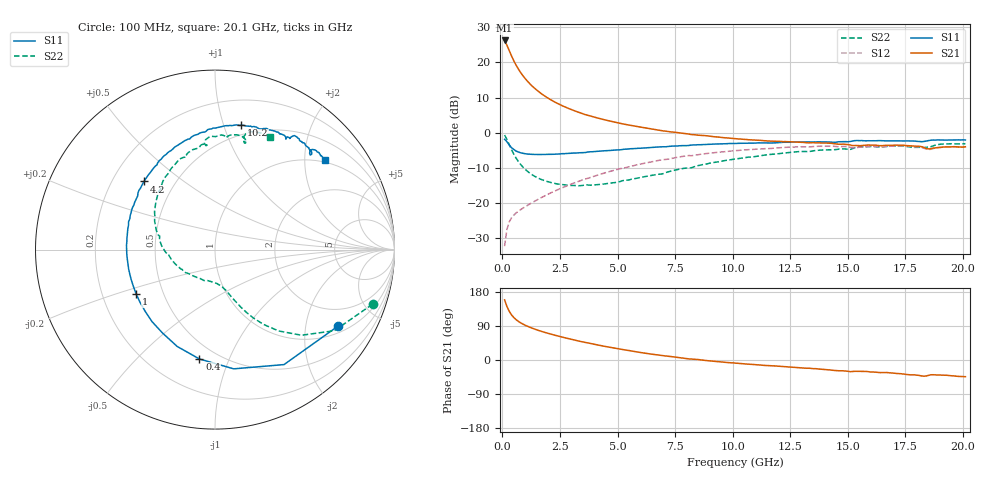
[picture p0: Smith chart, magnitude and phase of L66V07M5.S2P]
!  Infineon Technologies AG
! BFR380L3 , PF131585-7, No.6, Th 09.10.01, soldered on pcb-board, measured with PP GSG850
!  Vce=6.0 V,  Ic=7.5 mA
! Common Emitter S-Parameters:  15. November 2001
#  GHz  S  MA  R  50
! f  S11  S21  S12  S22
! GHz  Mag  Ang  Mag  Ang  Mag  Ang  Mag  Ang
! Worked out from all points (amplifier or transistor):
!   201 points, 100 MHz to 20.1 GHz, reference 50 ohm
!   highest |S21| = 26.2 dB at 100 MHz (marker M1)
!   |S21| within 3 dB of that: start of sweep to 307.7 MHz
!   unconditionally stable (mu >= 1): 2.049 GHz to 4.436 GHz
!   at 3.4 GHz: K = 1.04, MAG = 8.4 dB, |S12| = -13.6 dB
!   at 10.1 GHz: K = 0.93, MSG = 1.7 dB, |S12| = -5.1 dB
!   at 20.1 GHz: K = 0.99, MSG = 0.0 dB, |S12| = -4.0 dB
!   S11 on the Smith chart (normalised r, x): 100 MHz: 1.25, -3.05; 400 MHz: 0.40, -0.78; 1 GHz: 0.35, -0.23; 4.2 GHz: 0.34, +0.36; 10.2 GHz: 0.41, +1.14; 20.1 GHz: 0.95, +2.52
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0.1  0.8077 -31.8  20.44 158.5  0.02458 73.1  0.9288 -19.1
0.2  0.7472 -59.0  17.5 141.3  0.04233 62.2  0.8043 -34.2
0.3  0.6725 -81.1  14.67 128.6  0.05441 54.5  0.6781 -44.7
0.4  0.6154 -98.2  12.34 119.1  0.06205 50.2  0.5753 -52.0
0.5  0.5792 -111.4  10.51 112.0  0.06785 48.1  0.4965 -57.0
0.6  0.5489 -122.2  9.1 106.5  0.07287 47.2  0.4367 -60.7
0.7  0.5329 -131.3  8.012 101.8  0.07713 46.8  0.3902 -63.5
0.8  0.519 -138.7  7.131 97.9  0.08119 47.1  0.3538 -65.7
1  0.5039 -150.6  5.845 91.5  0.08951 48.2  0.3017 -69.0
1.2  0.4962 -159.9  4.945 86.2  0.09793 49.5  0.2668 -71.7
1.4  0.493 -167.6  4.288 81.7  0.1067 50.8  0.2417 -74.3
1.9  0.4936 177.4  3.23 71.9  0.1302 53.3  0.2058 -80.5
2.6  0.5058 162.1  2.422 60.4  0.1658 54.7  0.184 -91.4
3.5  0.523 146.2  1.859 47.6  0.2154 53.7  0.1792 -106.9
4.2  0.5477 136.1  1.6 38.9  0.2544 51.8  0.1845 -122.3
5.3  0.5848 122.2  1.324 26.7  0.317 46.6  0.2119 -144.6
6.8  0.6298 105.5  1.089 12.7  0.4066 37.9  0.2586 -173.1
10.1  0.7053 78.7  0.8248 -8.1  0.5564 15.9  0.4243 140.8
10.2  0.7083 78.2  0.8191 -8.7  0.5593 15.2  0.4289 139.5
13.5  0.7413 60.5  0.7239 -22.8  0.6371 -6.5  0.5543 106.4
16.8  0.7702 48.1  0.6625 -33.8  0.643 -23.6  0.6459 81.9
20.1  0.7903 38.9  0.6329 -44.0  0.6325 -37.7  0.6996 64.2
